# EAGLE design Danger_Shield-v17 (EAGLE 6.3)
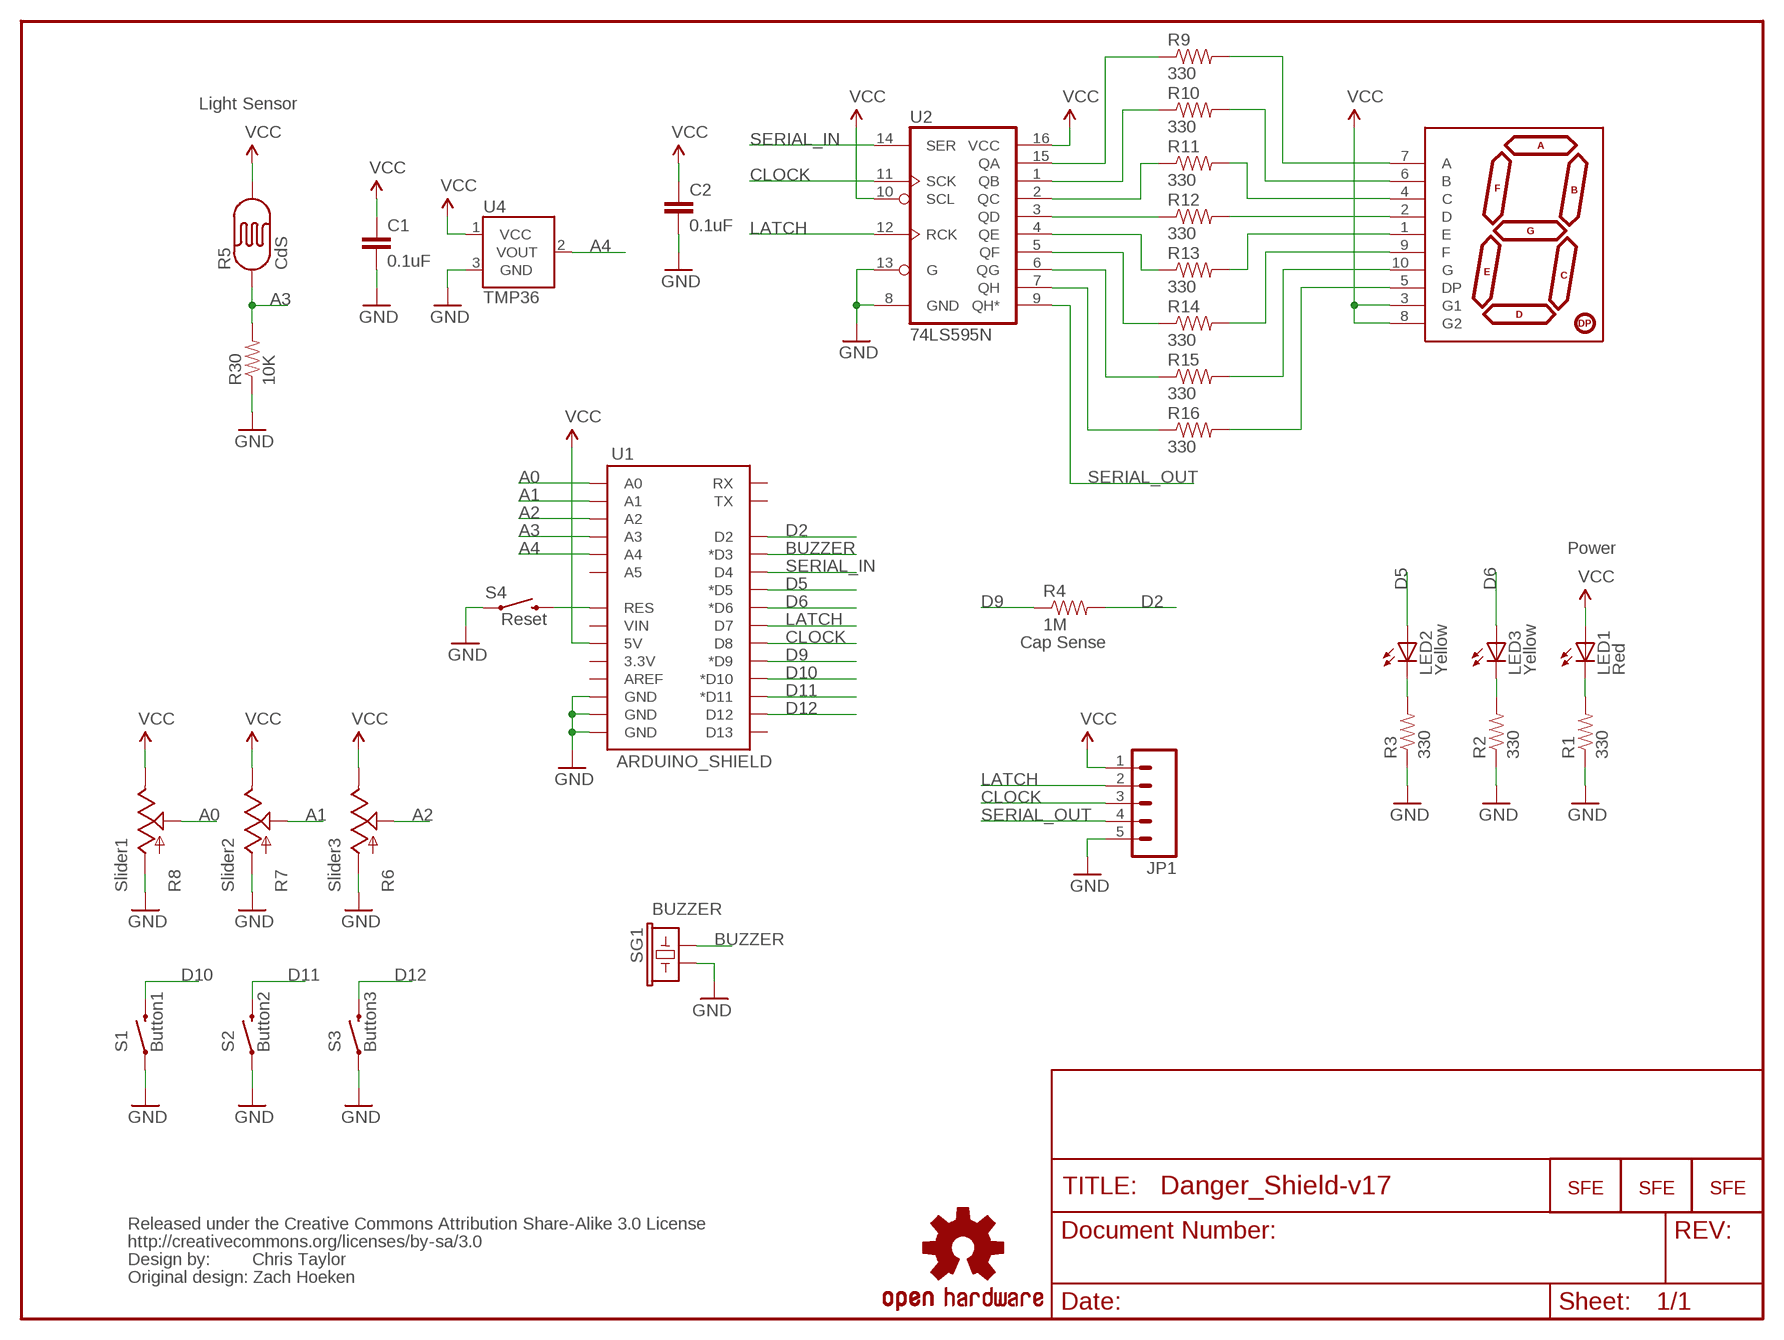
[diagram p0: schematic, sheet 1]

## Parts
C1  0.1uF  CAPPTH2  [CAP-PTH-SMALL2]
C2  0.1uF  CAPPTH2  [CAP-PTH-SMALL2]
JP1  M05PTH  [1X05]
JP2  LOGO-SFENEW  [SFE-NEW-WEBLOGO]
JP3  LOGO-SFENEW  [SFE-NEW-WEBLOGO]
JP5  LOGO-SFESK  [SFE-LOGO-FLAME]
LED1  Red  LED5MM  [LED5MM]
LED2  Yellow  LED5MM  [LED5MM]
LED3  Yellow  LED5MM  [LED5MM]
R1  330  RESISTORAXIAL-0.3  [AXIAL-0.3]
R2  330  RESISTORAXIAL-0.3  [AXIAL-0.3]
R3  330  RESISTORAXIAL-0.3  [AXIAL-0.3]
R4  1M  RESISTORAXIAL-0.3  [AXIAL-0.3]
R5  CdS  PHOTOCELLPTH  [PHOTOCELL]
R6  Slider3  SLIDER  [SLIDER]
R7  Slider2  SLIDER  [SLIDER]
R8  Slider1  SLIDER  [SLIDER]
R9  330  RESISTORAXIAL-0.3  [AXIAL-0.3]
R10  330  RESISTORAXIAL-0.3  [AXIAL-0.3]
R11  330  RESISTORAXIAL-0.3  [AXIAL-0.3]
R12  330  RESISTORAXIAL-0.3  [AXIAL-0.3]
R13  330  RESISTORAXIAL-0.3  [AXIAL-0.3]
R14  330  RESISTORAXIAL-0.3  [AXIAL-0.3]
R15  330  RESISTORAXIAL-0.3  [AXIAL-0.3]
R16  330  RESISTORAXIAL-0.3  [AXIAL-0.3]
R30  10K  RESISTORAXIAL-0.3  [AXIAL-0.3]
S1  Button1  SWITCH-MOMENTARY-212MM  [TACTILE-PTH-12MM]
S2  Button2  SWITCH-MOMENTARY-212MM  [TACTILE-PTH-12MM]
S3  Button3  SWITCH-MOMENTARY-212MM  [TACTILE-PTH-12MM]
S4  Reset  SWITCH-MOMENTARY-2PTH  [TACTILE-PTH]
SG1  BUZZER  BUZZERPTH  [BUZZER-12MM]
U1  ARDUINO_SHIELD  ARDUINO_SHIELDNO_SILK  [DUEMILANOVE_VIAS]
U2  74LS595N  [DIL16]
U4  TMP36  TMP36GT9  [TO-92]
U6  7-SEGMENT-DISPLAY-1"-RED  [7-SEGMENT-1"PTH]
U$1  CREATIVE_COMMONS  [CREATIVE_COMMONS]
U$2  OSHW-LOGOM  [OSHW-LOGO-M]

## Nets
A0: R8.2A(S) U1.A0
A1: R7.2A(S) U1.A1
A2: R6.2A(S) U1.A2
A3: R5.1 R30.P$2 U1.A3
A4: U1.A4 U4.2(VOUT)
BUZZER: SG1.+ U1.D3(*D3)
CLOCK: JP1.3 U1.D8 U2.11(SCK)
D2: R4.P$2 U1.D2
D5: LED2.A U1.D5(*D5)
D6: LED3.A U1.D6(*D6)
D9: R4.P$1 U1.D9(*D9)
D10: S1.3 U1.D10(*D10)
D11: S2.3 U1.D11(*D11)
D12: S3.3 U1.D12
GND: C1.2 C2.2 JP1.5 R1.P$1 R2.P$1 R3.P$1 R6.3(A) R7.3(A) R8.3(A) R30.P$1 S1.1 S2.1 S3.1 S4.1 SG1.- U1.GND@0(GND) U1.GND@1(GND) U1.GND@2(GND) U2.8(GND) U2.13(G) U4.3(GND)
LATCH: JP1.2 U1.D7 U2.12(RCK)
N$1: S4.3 U1.RES
N$2: R9.P$1 U2.15(QA)
N$3: LED1.K(C) R1.P$2
N$4: R10.P$1 U2.1(QB)
N$5: R11.P$1 U2.2(QC)
N$6: R12.P$1 U2.3(QD)
N$7: R13.P$1 U2.4(QE)
N$8: R14.P$1 U2.5(QF)
N$9: R15.P$1 U2.6(QG)
N$10: R16.P$1 U2.7(QH)
N$11: R9.P$2 U6.7(A)
N$12: R10.P$2 U6.6(B)
N$13: R11.P$2 U6.4(C)
N$14: R12.P$2 U6.2(D)
N$15: R13.P$2 U6.1(E)
N$16: R14.P$2 U6.9(F)
N$17: R15.P$2 U6.10(G)
N$18: R16.P$2 U6.5(DP)
N$19: LED3.K(C) R2.P$2
N$20: LED2.K(C) R3.P$2
SERIAL_IN: U1.D4 U2.14(SER)
SERIAL_OUT: JP1.4 U2.9(QH*)
VCC: C1.1 C2.1 JP1.1 LED1.A R5.2 R6.1(E) R7.1(E) R8.1(E) U1.5V U2.10(SCL) U2.16(VCC) U4.1(VCC) U6.3(G1) U6.8(G2)
Unconnected: U1.3.3V U1.A5 U1.AREF U1.D13 U1.RX U1.TX U1.VIN

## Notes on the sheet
- Light Sensor
- Power
- Cap Sense
- Chris Taylor
- Original design: Zach Hoeken

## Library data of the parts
C1 C2 = SparkFun-Passives:CAP: Capacitor
JP1 = SparkFun:M05: Header 5 Standard 5-pin 0.1" header. Use with straight break away headers (SKU : PRT-00116), right angle break away headers (PRT-00553), swiss pins (PRT-00743), machine pins (PRT-00117), and female headers (PRT-00115). Molex polarized connector foot print use with SKU : PRT-08230 with associated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
JP2 JP3 JP5 = SparkFun:LOGO-SFE: Spark Fun Electronics PCB Logo
LED1-LED3 = SparkFun:LED: LEDs
R1-R4 R9-R16 R30 = SparkFun:RESISTOR: Resistor
R5 = SparkFun:PHOTOCELL: Photocell Also known as a CdS photoresistor. This is a low cost way to detect light levels. Resistance decreases with more incoming light. SparkFun SKU: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
R6-R8 = SparkFun:SLIDER
S1-S4 = SparkFun:SWITCH-MOMENTARY-2
SG1 = SparkFun:BUZZER: Buzzer 12mm
U1 = SparkFun:ARDUINO_SHIELD
U2 = SparkFun:74*595: 8-bit SHIFT REGISTER, output latch
U4 = SparkFun-Sensors:TMP36: Precision degC temp sensor, analog out
U6 = SparkFun:7-SEGMENT-DISPLAY-1"-RED: 7-Segment Display 1" Red (COM-08546)
U$1 = SparkFun-Aesthetics:CREATIVE_COMMONS: Creative Commons License summary
U$2 = SparkFun-Aesthetics:OSHW-LOGO: Open Source Hardware Logo This logo indicates the piece of hardware it is found on incorporates a OSHW license and/or adheres to the definition of open source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

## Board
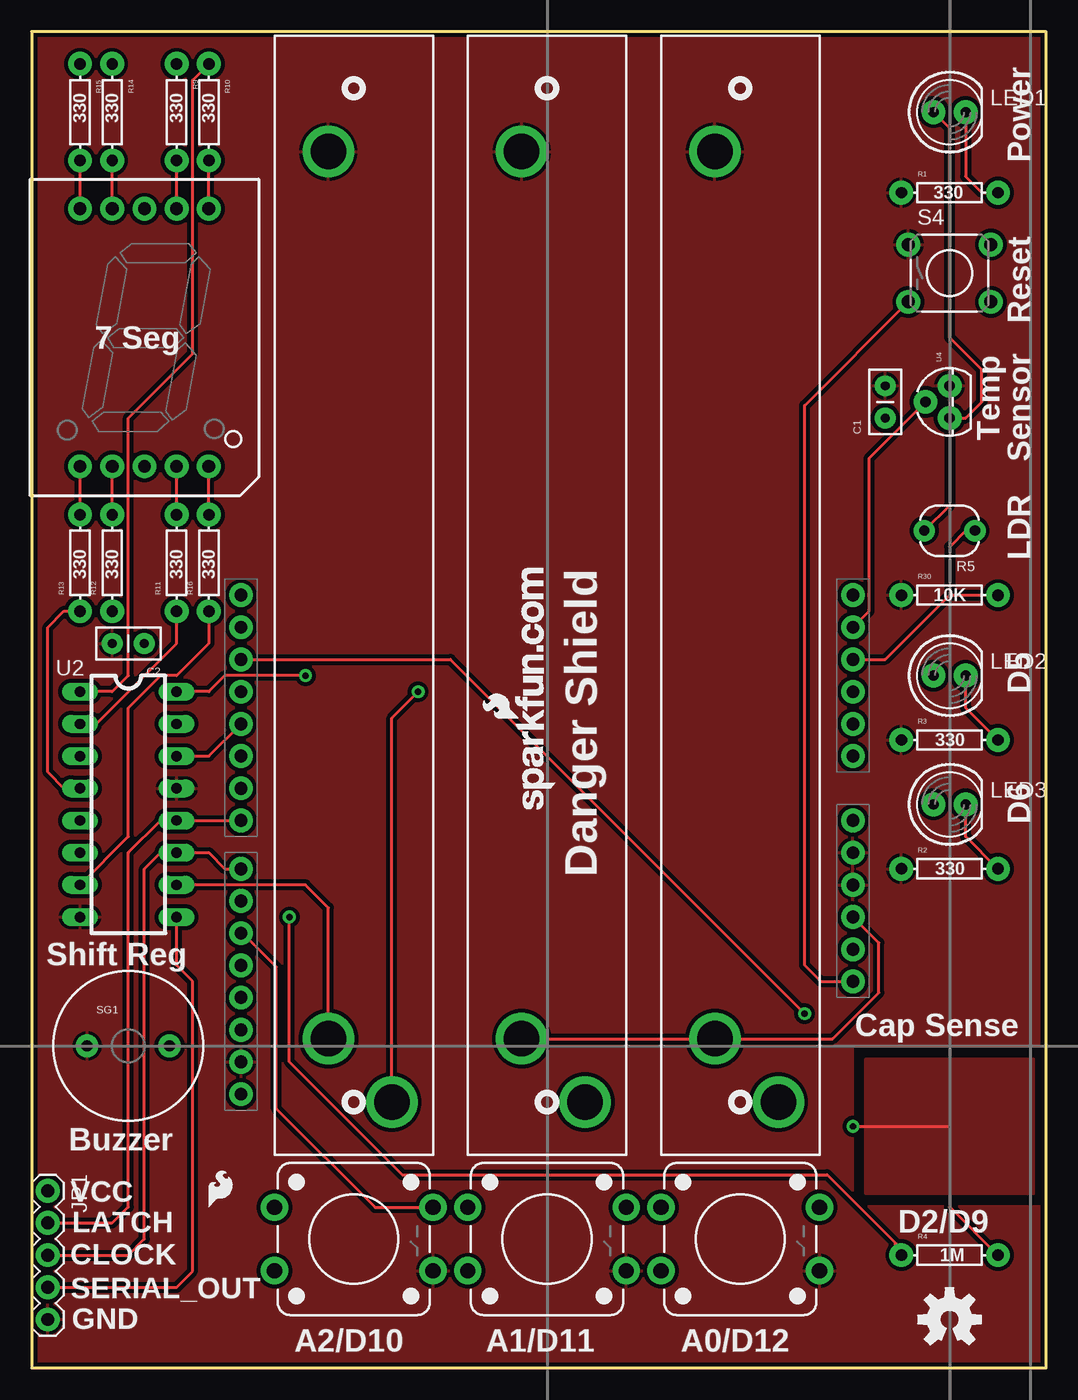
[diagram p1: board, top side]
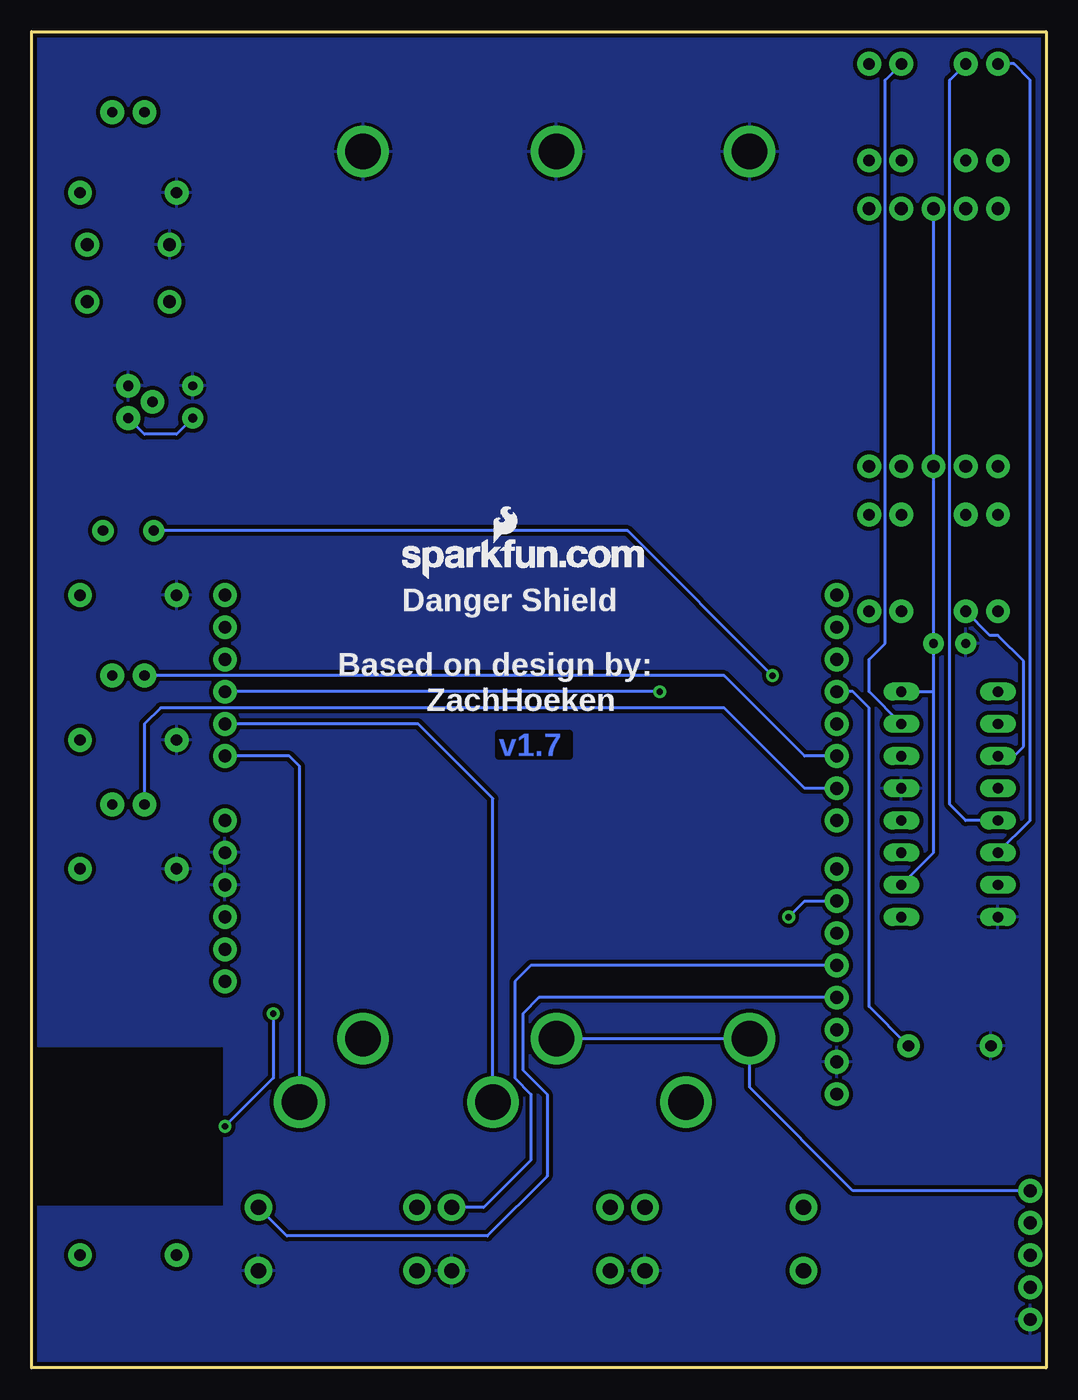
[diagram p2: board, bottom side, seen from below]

Size 80.01 x 105.41 mm. Coordinates in mm from the lower left corner, seen from the top.
Outline: 0,0 80.01,0 80.01,105.41 0,105.41 0,0
Copper layers (1*16): Top 0.035mm / dielectric 1.5mm / Bottom 0.035mm
Design rules "default": minimum track width 8mil, minimum drill 20mil, track to track 8mil, track to pad 8mil, pad to pad 8mil, via to via 8mil, smd to smd 8mil, copper to edge 8mil, drill to drill 8mil, minimum pad ring 12mil, minimum via ring 10mil, stop-mask expansion 4mil, vias tented up to drill 20mil, thermal gap 10mil

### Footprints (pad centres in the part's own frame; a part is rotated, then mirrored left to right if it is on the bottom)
CAP-PTH-SMALL2 = drill 0.7 pad 1.651: 1 0,0; 2 2.54,0
1X05 = drill 1.016 pad 1.88: 1 0,0; 2 2.54,0; 3 5.08,0; 4 7.62,0; 5 10.16,0
LED5MM = drill 0.813 pad 1.88: A -1.27,0; K 1.27,0
AXIAL-0.3 = drill 0.9 pad 1.88: P$1 -3.81,0; P$2 3.81,0
PHOTOCELL = drill 0.8 pad 1.676: 1 -2,0; 2 2,0
SLIDER = drill 2.8 pad 4.064: 1 -35,2; 2A -40,-3; 3 35,2
TACTILE-PTH-12MM = drill 1.2 pad 2.159: 1 6.25,-2.5; 2 -6.25,-2.5; 3 6.25,2.5; 4 -6.25,2.5
TACTILE-PTH = drill 1.016 pad 1.88: 1 -3.251,2.261; 2 3.251,2.261; 3 -3.251,-2.261; 4 3.251,-2.261
BUZZER-12MM = drill 0.9 pad 1.778: + 3.25,0; - -3.25,0
DUEMILANOVE_VIAS = drill 1.016 pad 1.88: 3.3V 50.8,13.97; 5V 50.8,16.51; A0 50.8,29.21; A1 50.8,31.75; A2 50.8,34.29; A3 50.8,36.83; A4 50.8,39.37; A5 50.8,41.91; AREF 2.54,2.54; D2 2.54,36.83; D3 2.54,34.29; D4 2.54,31.75; D5 2.54,29.21; D6 2.54,26.67; D7 2.54,24.13; D8 2.54,20.32; D9 2.54,17.78; D10 2.54,15.24; D11 2.54,12.7; D12 2.54,10.16; D13 2.54,7.62; GND@0 50.8,19.05; GND@1 50.8,21.59; GND@2 2.54,5.08; RES 50.8,11.43; RX 2.54,41.91; TX 2.54,39.37; VIN 50.8,24.13
DIL16 = drill 0.813 long: 1 -8.89,-3.81; 2 -6.35,-3.81; 3 -3.81,-3.81; 4 -1.27,-3.81; 5 1.27,-3.81; 6 3.81,-3.81; 7 6.35,-3.81; 8 8.89,-3.81; 9 8.89,3.81; 10 6.35,3.81; 11 3.81,3.81; 12 1.27,3.81; 13 -1.27,3.81; 14 -3.81,3.81; 15 -6.35,3.81; 16 -8.89,3.81
TO-92 = drill 0.813 pad 1.88: 1 -1.27,0; 2 0,1.905; 3 1.27,0
7-SEGMENT-1"PTH = drill 1 pad 1.88: 1 -5.08,-10.16; 2 -2.54,-10.16; 3 0,-10.16; 4 2.54,-10.16; 5 5.08,-10.16; 6 5.08,10.16; 7 2.54,10.16; 8 0,10.16; 9 -2.54,10.16; 10 -5.08,10.16

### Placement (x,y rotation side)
C1  67.31,74.93 90 top
C2  8.89,57.15 180 top
JP1  1.27,13.97 270 top
JP2  41.27,44.07 90 top
JP3  50.8,62.23 0 bottom
JP5  13.97,12.7 0 top
LED1  72.39,99.06 0 top
LED2  72.39,54.61 0 top
LED3  72.39,44.45 0 top
R1  72.39,92.71 0 top
R2  72.39,39.37 0 top
R3  72.39,49.53 0 top
R4  72.39,8.89 0 top
R5  72.39,66.04 180 top
R6  25.4,60.96 90 top
R7  40.64,60.96 90 top
R8  55.88,60.96 90 top
R9  11.43,99.06 270 top
R10  13.97,99.06 270 top
R11  11.43,63.5 90 top
R12  6.35,63.5 90 top
R13  3.81,63.5 90 top
R14  6.35,99.06 270 top
R15  3.81,99.06 270 top
R16  13.97,63.5 90 top
R30  72.39,60.96 0 top
S1  25.4,10.16 0 top
S2  40.64,10.16 0 top
S3  55.88,10.16 0 top
S4  72.39,86.36 0 top
SG1  7.62,25.4 0 top
U1  13.97,19.05 0 top
U2  7.62,44.45 270 top
U4  72.39,76.2 90 top
U6  8.89,81.28 0 top
U$1  not placed on the board
U$2  72.39,3.81 0 top

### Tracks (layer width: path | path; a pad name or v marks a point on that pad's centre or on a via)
A0
  Bottom 0.254: R8.2A 58.88,47.45 59.69,48.26 U1.A0
A1
  Bottom 0.254: R7.2A 43.64,44.91 49.53,50.8 U1.A1
A2  (via drill 0.51)
  Top 0.254: R6.2A 28.4,51.26 v30.48,53.34
  Bottom 0.254: v30.48,53.34 U1.A2
A3
  Top 0.254: 72.39,60.96 67.31,55.88 U1.A3 | R5.1 73.66,66.04 72.39,64.77 72.39,60.96 | 72.39,60.96 R30.P$2
A4
  Top 0.254: U1.A4 66.04,59.69 66.04,71.75 U4.2
BUZZER
  Bottom 0.254: U1.D3 15.24,53.34 13.97,52.07 13.97,28.5 SG1.+
CLOCK
  Top 0.254: U1.D8 15.24,39.37 13.97,40.64 U2.11 10.16,40.64 8.89,39.37 8.89,10.16 7.62,8.89 JP1.3
D2  (via drill 0.51)
  Top 0.254: U1.D2 33.02,55.88 v60.96,27.94 | v64.77,19.05 72.39,19.05 72.39,12.7 R4.P$2
  Bottom 0.254: v60.96,27.94 60.96,22.86 v64.77,19.05
  pour Top: 65.79,24.38 78.99,24.38 78.99,13.72 65.79,13.72
D5
  Bottom 0.254: LED2.A 25.4,54.61 19.05,48.26 U1.D5
D6
  Bottom 0.254: U1.D6 19.05,45.72 25.4,52.07 69.85,52.07 71.12,50.8 LED3.A
D9  (via drill 0.51)
  Top 0.254: 68.2,9.78 68.07,9.78 | 68.2,9.78 62.74,15.24 29.21,15.24 20.32,24.13 v20.32,35.56 | R4.P$1 68.58,9.4 68.2,9.78
  Bottom 0.254: v20.32,35.56 19.05,36.83 U1.D9
D10
  Top 0.254: S1.3 27.09,12.66 19.3,20.45 19.3,31.62 16.64,34.29 U1.D10
D11
  Bottom 0.254: U1.D11 40.64,31.75 41.91,30.48 41.91,22.86 40.64,21.59 40.64,16.38 44.36,12.66 S2.3
D12
  Bottom 0.254: U1.D12 40.01,29.21 41.27,27.94 41.27,23.5 39.37,21.59 39.37,15.11 44.07,10.41 59.88,10.41 S3.3
GND
  pour Top (isolate 0.305): 0,105.41 0,0 80.01,0 80.01,12.7 64.77,12.7 64.77,25.4 80.01,25.4 80.01,105.41
  pour Bottom (isolate 0.305): 0,105.41 0,0 80.01,0 80.01,12.7 64.77,12.7 64.77,25.4 80.01,25.4 80.01,105.41
LATCH
  Top 0.254: U1.D7 U2.12 10.16,43.18 7.62,40.64 7.62,12.7 6.35,11.43 JP1.2
N$1
  Top 0.254: U1.RES 62.23,30.48 60.96,31.75 60.96,75.92 S4.3
N$2
  Bottom 0.254: R9.P$1 12.7,101.6 12.7,57.15 13.97,55.88 13.97,53.34 U2.15
N$3
  Top 0.254: LED1.K 73.66,93.98 74.93,92.71 R1.P$2
N$4
  Top 0.254: R10.P$1 12.7,101.6 12.7,80.01 7.62,74.93 7.62,54.61 6.35,53.34 U2.1
N$5
  Top 0.254: U2.2 5.08,50.8 11.43,57.15 R11.P$1
N$6
  Bottom 0.254: U2.3 2.54,48.26 1.78,49.02 1.78,55.75 3.81,57.78 4.45,57.78 R12.P$1
N$7
  Top 0.254: R13.P$1 2.54,59.69 1.27,58.42 1.27,46.99 2.54,45.72 U2.4
N$8
  Bottom 0.254: R14.P$1 7.62,101.6 7.62,44.45 6.35,43.18 U2.5
N$9
  Bottom 0.254: R15.P$1 2.54,102.87 1.27,101.6 1.27,43.18 U2.6
N$10
  Top 0.254: U2.7 7.62,41.91 7.62,52.07 10.16,54.61 11.43,54.61 13.97,57.15 R16.P$1
N$11
  Top 0.254: U6.7 R9.P$2
N$12
  Top 0.254: U6.6 R10.P$2
N$13
  Top 0.254: R11.P$2 U6.4
N$14
  Top 0.254: R12.P$2 U6.2
N$15
  Top 0.254: R13.P$2 U6.1
N$16
  Top 0.254: U6.9 R14.P$2
N$17
  Top 0.254: U6.10 R15.P$2
N$18
  Top 0.254: R16.P$2 U6.5
N$19
  Top 0.254: LED3.K 73.66,41.91 R2.P$2
N$20
  Top 0.254: LED2.K 73.66,52.07 R3.P$2
SERIAL_IN
  Top 0.254: U2.14 13.97,48.26 U1.D4
SERIAL_OUT
  Top 0.254: U2.9 11.43,31.75 12.7,30.48 12.7,7.62 11.43,6.35 JP1.4
VCC  (via drill 0.51)
  Top 0.254: R7.1 R8.1 63.17,25.96 66.8,29.59 66.8,33.53 U1.5V | U2.10 21.59,38.1 23.4,36.29 R6.1 | R5.2 72.39,68.04 U4.1 73.66,74.93 74.93,76.2 74.93,78.74 72.39,81.28 72.39,97.79 LED1.A | v21.59,54.61 15.24,54.61 13.97,53.34 U2.16
  Bottom 0.254: R7.1 R6.1 23.4,22.13 15.24,13.97 JP1.1 | 8.89,53.34 8.89,40.64 U2.10 | 8.89,53.34 C2.1 U6.3 U6.8 | v21.59,54.61 33.02,66.04 R5.2 | U2.16 8.89,53.34 | C1.1 68.58,73.66 71.12,73.66 U4.1

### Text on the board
Bottom: v1.7
tPlace: Power | Reset | 7 Seg | Temp | Sensor | LDR | D5 | D6 | Danger Shield | Shift Reg | Cap Sense | Buzzer | VCC | LATCH | D2/D9 | CLOCK | SERIAL_OUT | GND | A2/D10 | A1/D11 | A0/D12 | Chris Taylor
bPlace: Danger Shield | Based on design by: | ZachHoeken
Measures: 4150 | 0 | 0 | All Dimensions in mil | Spark Fun Electronics | 0 | 0 | 3150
